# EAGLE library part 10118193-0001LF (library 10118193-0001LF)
USB Connectors 5P MICRO USB TYPE B RECEPTACLE W/ PEGS Source: Datasheet
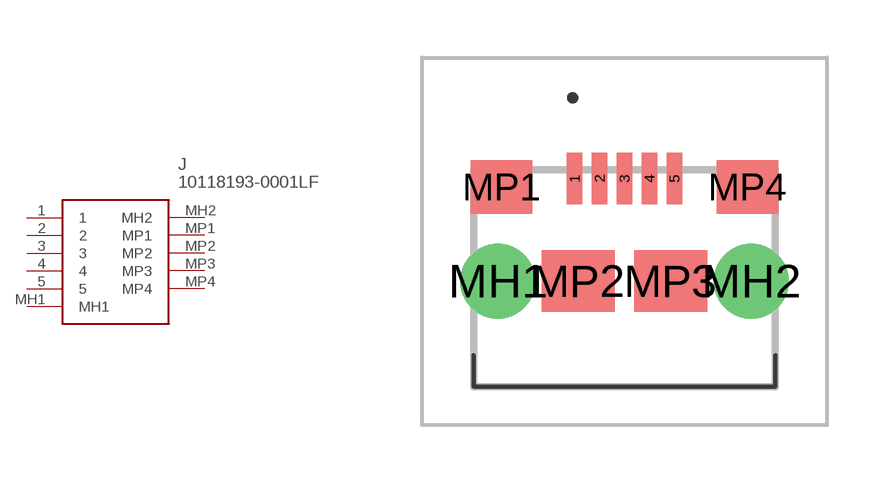
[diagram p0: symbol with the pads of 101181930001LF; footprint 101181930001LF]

Designator prefix J

## 10118193-0001LF (Arrow_Part_Number: 10118193-0001LF; Arrow_Price-Stock: https://www.arrow.com/en/products/10118193-0001lf/amphenol-fci?region=nac; Description: USB Connectors 5P MICRO USB TYPE B RECEPTACLE W/ PEGS; Height: 3.1mm; Manufacturer_Name: Amphenol; Manufacturer_Part_Number: 10118193-0001LF; Mouser_Part_Number: 649-10118193-0001LF; Mouser_Price-Stock: https://www.mouser.co.uk/ProductDetail/Amphenol-FCI/10118193-0001LF?qs=Ywefl8B65e63Nsqd%252B8HZaQ%3D%3D)  [101181930001LF]
1  1
2  2
3  3
4  4
5  5
MH1  MH1
MH2  MH2
MP1  MP1
MP2  MP2
MP3  MP3
MP4  MP4

## Footprint 101181930001LF (pad centres in mm)
10118193-0001LF-1
smd 0.4 x 1.35: 1 -1.3,2.6; 2 -0.65,2.6; 3 0,2.6; 4 0.65,2.6; 5 1.3,2.6
drill 1.3 pad 1.95: MH1 -3.3,-0.075; MH2 3.3,-0.075
smd 1.6 x 1.4: MP1 -3.2,2.375; MP4 3.2,2.375
smd 1.9 x 1.6: MP2 -1.2,-0.075; MP3 1.2,-0.075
